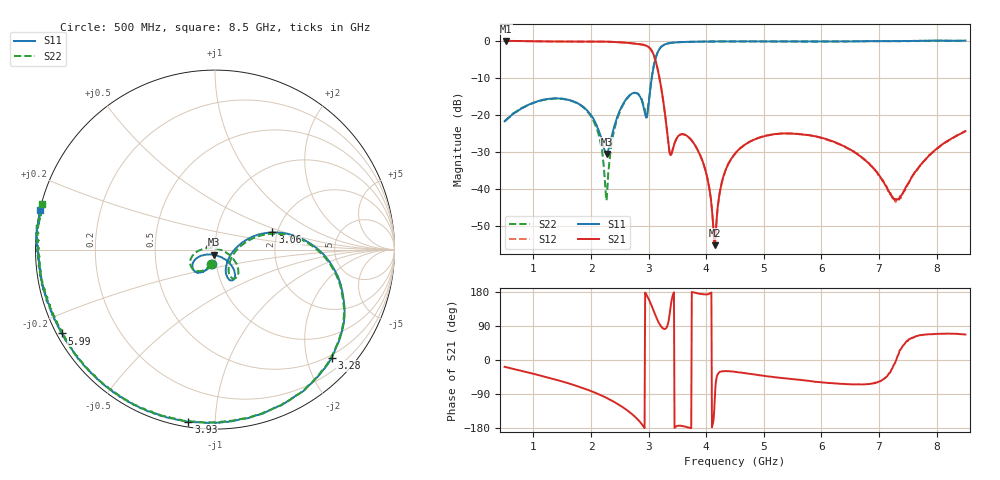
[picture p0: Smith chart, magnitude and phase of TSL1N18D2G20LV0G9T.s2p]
! TSL1N18D2G20LV0G9T  S-PARAMETER MODEL  ( General Type )
! Model Generated by TAIYO YUDEN Corporation (https://www.yuden.co.jp/en/)
! Version 1.0
! TAIYO YUDEN Control No. 131002
! Copyright(c) 2013 TAIYO YUDEN CO.,LTD. All Rights Reserved.
! Products Name : Multilayer Ceramic Devices
! Characteristics :
!  Passband freq : 1700-2170MHz,2170-2500MHz,2500-2700MHz ( At Passband , Insertion Loss : 0.55dB,0.75dB,1.0dB , VSWR 1.92 ),
!  Attenuation : 25dB min at 3400MHz, 22dB min at 3400-5400MHz, 20dB min at 5400-8100MHz , Impedance : 50 Ohm ,
!  Case Size : 1.6 x 0.8 / 0.063 x 0.031 [mm/inch] , Thickness : 0.45 / 0.018 [mm/inch]
!  (Conditions: Temperature = 25 degC , DC Bias Current/Voltage = 0A / 0V)
! External Node Assignments :
!  1  o---|-------|---o  2
!  |  LPF  |
! GND o---|-------|---o GND
! Frequency Range : 500MHz  -  8.5GHz  [ 801 STEP ]
# MHz S RI R 50
! Freq[MHz].  S11 Real  S11 Imag  S21 Real  S21 Imag  S12 Real  S12 Imag  S22 Real  S22 Imag
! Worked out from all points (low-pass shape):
!   801 points, 500 MHz to 8.5 GHz, reference 50 ohm
!   highest |S21| = -0.07 dB at 520 MHz (marker M1); lowest = -55.3 dB at 4.15 GHz (marker M2)
!   |S21| within 3 dB of the highest: start of sweep to 3.065 GHz
!   lowest |S11| = -30.6 dB at 2.27 GHz (marker M3), VSWR 1.06, Z = 49.3 - j2.85 ohm
!   |S11| at or under -10 dB: start of sweep to 3.056 GHz
!   |S22| runs from -43.2 to 0.0 dB; largest |S21 - S12| = 0.0023
!   S11 on the Smith chart (normalised r, x): 500 MHz: 0.96, -0.15; 3.06 GHz: 1.88, +0.41; 3.28 GHz: 0.44, -2.48; 3.93 GHz: 0.03, -0.86; 5.99 GHz: 0.01, -0.26; 8.5 GHz: -0.00, +0.11
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500  -0.0161 -0.0796  0.9431 -0.3057  0.9426 -0.305  -0.0214 -0.0788
520  -0.0177 -0.0817  0.9394 -0.3175  0.9388 -0.3164  -0.0232 -0.0811
1840  -0.1158 -0.062  0.2841 -0.926  0.284 -0.9255  -0.1254 -0.0343
2110  -0.0601 -0.0295  0.0204 -0.9685  0.0211 -0.9674  -0.0611 0.005
2270  -0.00573 -0.0289  -0.1685 -0.952  -0.1676 -0.9509  0.00141 0.00678
2510  0.0859 -0.0811  -0.4803 -0.8165  -0.4808 -0.817  0.1014 -0.051
2770  0.0972 -0.1707  -0.7914 -0.4451  -0.7917 -0.4462  0.1164 -0.158
2960  0.0778 -0.0465  -0.8457 0.1052  -0.8453 0.1043  0.0906 -0.0477
3060  0.3197 0.0962  -0.5502 0.453  -0.5504 0.453  0.3266 0.0886
3170  0.7002 -0.1938  -0.0666 0.363  -0.0656 0.3625  0.6988 -0.2032
3280  0.6494 -0.6035  0.0155 0.1084  0.0156 0.1081  0.6412 -0.6119
3380  0.4791 -0.7973  -0.0211 0.0191  -0.021 0.0192  0.4668 -0.8042
3620  0.1407 -0.9445  -0.0537 -0.00467  -0.0535 -0.00452  0.1163 -0.9479
3930  -0.1482 -0.9596  -0.0242 0.0025  -0.0243 0.00273  -0.1818 -0.9526
4150  -0.2918 -0.9283  -0.000318 -0.00169  -0.000209 -0.00166  -0.3276 -0.9128
4290  -0.3658 -0.9018  0.012 -0.00672  0.0119 -0.00678  -0.4051 -0.8842
4500  -0.4635 -0.8573  0.0253 -0.0154  0.0253 -0.0155  -0.5018 -0.8328
5840  -0.8267 -0.5105  0.0288 -0.043  0.0297 -0.0428  -0.85 -0.4692
5990  -0.8532 -0.467  0.0256 -0.0418  0.0256 -0.0414  -0.8739 -0.4259
7170  -0.9771 -0.1183  0.00749 -0.00547  0.00735 -0.00544  -0.9763 -0.0874
7330  -0.9786 -0.0721  0.00703 0.00152  0.00684 0.0016  -0.9833 -0.0429
8500  -0.9756 0.2202  0.0231 0.055  0.023 0.0557  -0.9649 0.2542
